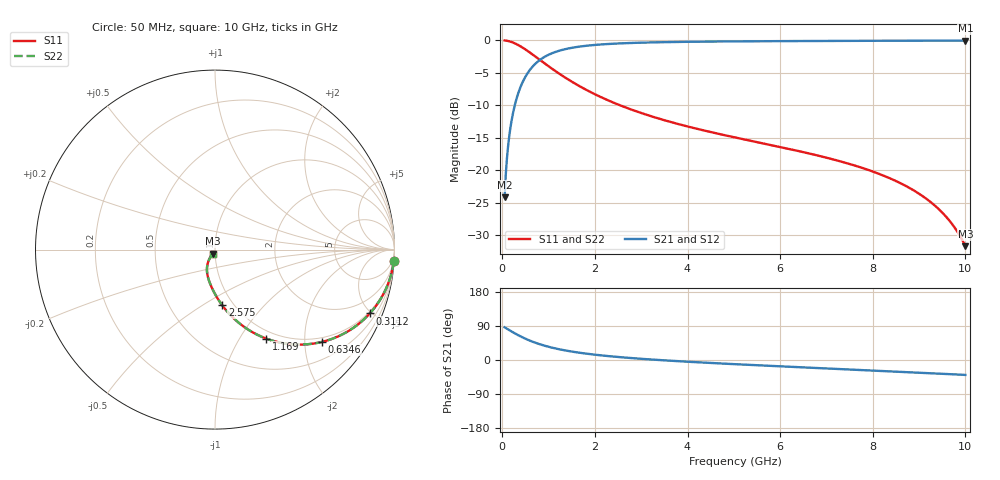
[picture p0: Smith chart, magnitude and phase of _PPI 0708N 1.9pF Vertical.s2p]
! S-Parameter data specifications (vertical orientation):
! Substrate: 40-mil Rogers 3003C, Substrate thickness, H=1.016mm, Dielectric constant, Er=3, Conductor thickness, T_mtl=0.043mm, Loss Tangent, Tand=0.003
! PCB Mounting Pad Footprint: Pad width, PadW=2.54mm , Pad length, PadL=0.51mm , Pad gap, PadG (edge-to-edge)=0.71mm , Reference planes=1.73mm apart
! Created Tue Jan 16 08:44:02 2018
# GHz S MA R 50
! 2 Port Network Data from SP1.SP block
! freq  magS11  angS11  magS21  angS21  magS12  angS12  magS22  angS22
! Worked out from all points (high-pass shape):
!   801 points, 50 MHz to 10 GHz, reference 50 ohm
!   highest |S21| = -0.04 dB at 10 GHz (marker M1); lowest = -24.2 dB at 50 MHz (marker M2)
!   |S21| within 3 dB of the highest: 807.5 MHz to end of sweep
!   lowest |S11| = -31.7 dB at 10 GHz (marker M3), VSWR 1.05, Z = 48.6 - j2.18 ohm
!   |S11| at or under -10 dB: 2.541 GHz to end of sweep
!   |S22| runs from -31.7 to 0.0 dB; largest |S21 - S12| = 0
!   S11 on the Smith chart (normalised r, x): 50 MHz: 1, -30; 311.2 MHz: 0.89, -4.90; 634.6 MHz: 0.89, -2.41; 1.169 GHz: 0.89, -1.31; 2.575 GHz: 0.89, -0.61; 10 GHz: 0.97, -0.04
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0.05  0.9981 -3.8  0.06175 86.2  0.06175 86.2  0.9981 -3.8
0.074875  0.9957 -5.6  0.09225 84.4  0.09225 84.4  0.9957 -5.6
0.124625  0.9883 -9.3  0.1524 80.7  0.1524 80.7  0.9883 -9.3
0.174375  0.9775 -12.9  0.2109 77.1  0.2109 77.1  0.9775 -12.9
0.2365625  0.9597 -17.3  0.2808 72.7  0.2808 72.7  0.9597 -17.3
0.3111875  0.9332 -22.4  0.3591 67.6  0.3591 67.6  0.9332 -22.4
0.448  0.8748 -30.9  0.4841 59.1  0.4841 59.1  0.8748 -30.9
0.6345625  0.7873 -40.8  0.6161 49.2  0.6161 49.2  0.7873 -40.8
0.89575  0.672 -51.6  0.7399 38.4  0.7399 38.4  0.672 -51.6
1.169375  0.5725 -60.0  0.8191 29.9  0.8191 29.9  0.5725 -60.0
1.418125  0.5009 -66.0  0.8646 23.9  0.8646 23.9  0.5009 -66.0
1.716625  0.4338 -71.6  0.9 18.3  0.9 18.3  0.4338 -71.6
2.574813  0.3128 -82.6  0.9485 7.2  0.9485 7.2  0.3128 -82.6
3.370812  0.2503 -89.6  0.9667 0.1  0.9667 0.1  0.2503 -89.6
5.025  0.1787 -100.5  0.9819 -11.0  0.9819 -11.0  0.1787 -100.5
6.691625  0.1328 -109.5  0.9886 -20.5  0.9886 -20.5  0.1328 -109.5
7.624437  0.1082 -114.2  0.9912 -25.6  0.9912 -25.6  0.1082 -114.2
8.345812  0.08732 -117.7  0.9929 -29.6  0.9929 -29.6  0.08732 -117.7
8.893062  0.06956 -120.1  0.994 -32.7  0.994 -32.7  0.06956 -120.1
9.340813  0.05335 -121.6  0.9947 -35.3  0.9947 -35.3  0.05335 -121.6
9.689063  0.03946 -122.0  0.9951 -37.5  0.9951 -37.5  0.03946 -122.0
10  0.02598 -120.6  0.9953 -39.4  0.9953 -39.4  0.02598 -120.6
